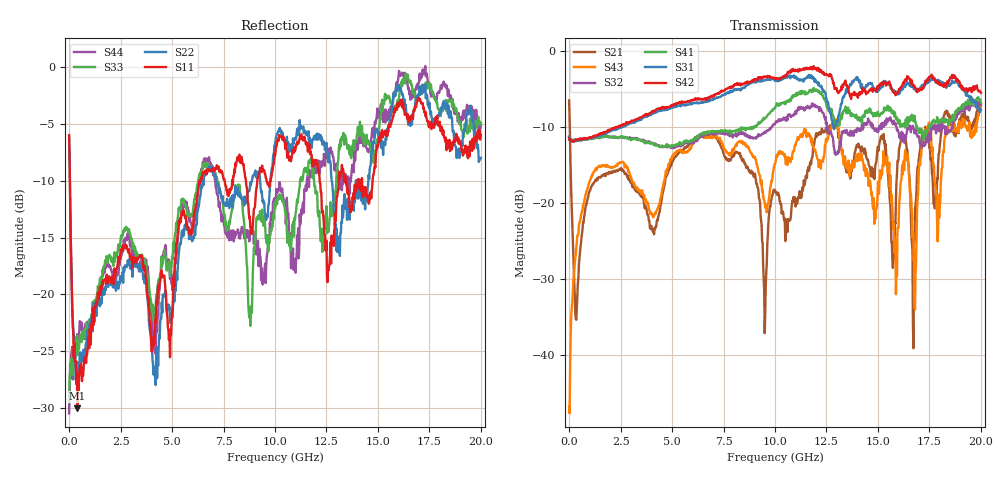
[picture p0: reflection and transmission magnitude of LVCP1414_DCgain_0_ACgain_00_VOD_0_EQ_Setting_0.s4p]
!Agilent Technologies,N5230A,MY46400459,A.07.50.48
!Agilent N5230A: A.07.50.48
!Date: Tuesday, April 17, 2012 18:33:27
!Correction: S11(Full 4 Port(1,2,3,4))
!S12(Full 4 Port(1,2,3,4))
!S13(Full 4 Port(1,2,3,4))
!S14(Full 4 Port(1,2,3,4))
!S21(Full 4 Port(1,2,3,4))
!S22(Full 4 Port(1,2,3,4))
!S23(Full 4 Port(1,2,3,4))
!S24(Full 4 Port(1,2,3,4))
!S31(Full 4 Port(1,2,3,4))
!S32(Full 4 Port(1,2,3,4))
!S33(Full 4 Port(1,2,3,4))
!S34(Full 4 Port(1,2,3,4))
!S41(Full 4 Port(1,2,3,4))
!S42(Full 4 Port(1,2,3,4))
!S43(Full 4 Port(1,2,3,4))
!S44(Full 4 Port(1,2,3,4))
!S4P File: Measurements: <S11,S12,S13,S14>,
!<S21,S22,S23,S24>,
!<S31,S32,S33,S34>,
!<S41,S42,S43,S44>:
# Hz S  dB  R 50
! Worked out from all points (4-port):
!   801 points, 300 kHz to 20 GHz, reference 50 ohm
!   strongest paths, dB at 300 kHz, 5 GHz, 10 GHz, 15 GHz, 20 GHz:
!     S42: -11.4, -7.1, -3.6, -4.7, -5.5
!     S31: -11.2, -7.4, -3.9, -5.3, -7.7
!     S41: -11.3, -12.4, -7.5, -8.0, -6.8
!     S32: -11.4, -12.7, -9.5, -10.6, -6.9
!     S43: -46.8, -13.9, -14.8, -17.2, -7.3
!     S21: -6.5, -14.6, -18.5, -12.6, -7.1
!   lowest |S11| = -30.0 dB at 400.3 MHz (marker M1), VSWR 1.07, Z = 52.9 + j1.4 ohm
!   |S11| at or under -10 dB: 37.57 MHz to 6.371 GHz (6.333 GHz wide, 198 % of centre); 8.585 GHz to 9.142 GHz (557.1 MHz wide, 6.29 % of centre); 12.17 GHz to 13.1 GHz (928.5 MHz wide, 7.35 % of centre)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
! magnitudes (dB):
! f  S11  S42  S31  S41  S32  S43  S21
! 300 kHz  -6.0  -11.4  -11.2  -11.3  -11.4  -46.8  -6.5
! 400.3 MHz  -30.0  -11.6  -11.7  -11.7  -11.7  -24.2  -32.2
! 10.05 GHz  -7.1  -3.6  -3.9  -7.2  -9.2  -14.2  -18.5
! 12.75 GHz  -14.8  -3.4  -9.0  -7.6  -11.0  -9.8  -10.1
! 14.05 GHz  -10.7  -5.7  -3.7  -8.7  -10.3  -13.5  -12.2
! 16.78 GHz  -3.8  -4.8  -4.7  -8.5  -10.8  -33.2  -25.2
! 20 GHz  -6.0  -5.5  -7.7  -6.8  -6.9  -7.3  -7.1
